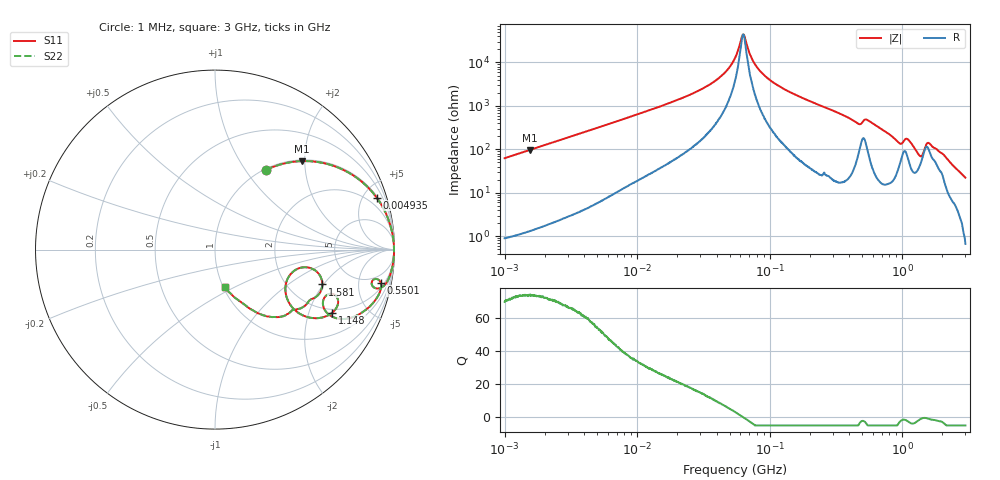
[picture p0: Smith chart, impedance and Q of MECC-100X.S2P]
!s-Parameter Generated by FASTRON Sdn. Bhd.
!FASTRON P/N : MECC-100X
!Keysight Technologies,E4991B,MY54100416,A.01.15
!Date: Thu Aug 20 13:09:35 2026
!Version  : Rev00 Thu Aug 20 13:09:35 2026
!Data & Calibration Information:
!PortZ  Port1:50+j0  Port2:50+j0
!When reading, reference impedance value at option line is always used.
!Remarks : This data is being provided solely for informational purposes.
!Freq	S11	S21	S12	S22
# Hz S dB R 50
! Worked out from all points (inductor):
!   1601 points, 1 MHz to 3 GHz, reference 50 ohm
!   read as one part in series: L = 9.95 uH near 1.041 MHz
!   highest Q = 73.8 at 1.545 MHz (marker M1), where L = 9.95 uH
!   self-resonance near 63.01 MHz
!   S11 on the Smith chart (normalised r, x): 1 MHz: 1.02, +1.25; 4.935 MHz: 1.11, +6.18; 550.1 MHz: 2.77, -9.21; 1.148 GHz: 1.83, -2.87; 1.581 GHz: 3.03, -1.95; 3 GHz: 1.01, -0.45
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1000000  -5.56 57.4  -1.49 -31.8  -1.49 -31.8  -5.56 57.4
1545498  -3.22 45.6  -2.92 -43.7  -2.92 -43.7  -3.22 45.6
3804036  -0.76 22.7  -8.28 -66.4  -8.28 -66.4  -0.76 22.7
4934590  -0.48 17.8  -10.27 -71.1  -10.27 -71.1  -0.48 17.8
1.447069e7  -0.08 6.0  -19.54 -81.8  -19.54 -81.8  -0.08 6.0
3.597591e7  -0.03 1.8  -30.20 -83.3  -30.20 -83.3  -0.03 1.8
4.643495e7  -0.02 0.9  -35.64 -80.5  -35.64 -80.5  -0.02 0.9
5.477226e7  -0.02 0.4  -42.04 -72.1  -42.04 -72.1  -0.02 0.4
6.364388e7  -0.02 -0.0  -52.90 9.0  -52.90 9.0  -0.02 -0.0
7.46963e7  -0.02 -0.5  -40.89 75.3  -40.89 75.3  -0.02 -0.5
9.034013e7  -0.02 -1.1  -34.32 82.7  -34.32 82.7  -0.02 -1.1
2.083556e8  -0.05 -4.6  -21.84 83.8  -21.84 83.8  -0.05 -4.6
4.616833e8  -0.60 -13.4  -12.55 66.9  -12.55 66.9  -0.60 -13.4
5.500551e8  -0.52 -11.4  -13.94 67.7  -13.94 67.7  -0.52 -11.4
7.925923e8  -0.99 -23.1  -8.12 62.8  -8.12 62.8  -0.99 -23.1
9.682285e8  -3.23 -28.3  -5.83 39.7  -5.83 39.7  -3.23 -28.3
1.147801e9  -2.60 -28.4  -6.09 45.4  -6.09 45.4  -2.60 -28.4
1.360679e9  -6.73 -31.4  -3.71 21.6  -3.71 21.6  -6.73 -31.4
1.466741e9  -6.02 -11.4  -5.70 11.0  -5.70 11.0  -6.02 -11.4
1.581072e9  -4.03 -18.0  -7.00 25.7  -7.00 25.7  -4.03 -18.0
2.134733e9  -5.98 -48.4  -2.33 29.4  -2.33 29.4  -5.98 -48.4
3e9  -13.29 -75.8  -0.27 12.5  -0.27 12.5  -13.29 -75.8
